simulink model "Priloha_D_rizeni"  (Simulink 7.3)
settings: Solver=ode45  StartTime=0.0  StopTime=0.7  FixedStep=0.6e-3  MaxStep=0.08e-3  RelTol=0.8e-3
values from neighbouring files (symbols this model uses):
  ILi = [0 Imax]    [Priloha_B_motor1_parametry.m]    (also in Priloha_C_motor2_parametry.m)
  Im = Psim / Ldi(1)    [Priloha_B_motor1_parametry.m]    (also in Priloha_C_motor2_parametry.m)
  Imax = 8    [Priloha_B_motor1_parametry.m]    (also in Priloha_C_motor2_parametry.m)
  J = 7e-3    (= 0.007)    [Priloha_B_motor1_parametry.m]    (also in Priloha_C_motor2_parametry.m)
  Kiid = 1 / (KM * 2 * tausigmaid / Rs)    (= 1975)    [Priloha_B_motor1_parametry.m]    (also in Priloha_C_motor2_parametry.m)
  Kiiq = 1 / (KM * 2 * tausigmaiq / Rs)    (= 1975)    [Priloha_B_motor1_parametry.m]    (also in Priloha_C_motor2_parametry.m)
  Kiwq = 1 / (Psim * p * 8 * (2 * tausigmaiq)^2 / J)    (= 306.115309264)    [Priloha_B_motor1_parametry.m]    (also in Priloha_C_motor2_parametry.m = 402.854511971)
  KM = 1    [Priloha_B_motor1_parametry.m]    (also in Priloha_C_motor2_parametry.m)
  Kpid = Ldi(1) / (KM * 2 * tausigmaid)    [Priloha_B_motor1_parametry.m]    (also in Priloha_C_motor2_parametry.m)
  Kpiq = Lqi(1) / (KM * 2 * tausigmaiq)    [Priloha_B_motor1_parametry.m]    (also in Priloha_C_motor2_parametry.m)
  Kpwq = 4 / (Psim * p * 8 * (2 * tausigmaiq) / J)    (= 2.44892247411)    [Priloha_B_motor1_parametry.m]    (also in Priloha_C_motor2_parametry.m = 3.22283609576)
  Ld = 22.5e-3    (= 0.0225)    [Priloha_B_motor1_parametry.m]    (also in Priloha_C_motor2_parametry.m)
  Ldi = [Ldi Ldi]    [Priloha_B_motor1_parametry.m]    (also in Priloha_C_motor2_parametry.m)
  Lq = 54e-3    (= 0.054)    [Priloha_B_motor1_parametry.m]    (also in Priloha_C_motor2_parametry.m)
  Lqi = [Lqi Lqi]    [Priloha_B_motor1_parametry.m]    (also in Priloha_C_motor2_parametry.m)
  p = 3    [Priloha_B_motor1_parametry.m]    (also in Priloha_C_motor2_parametry.m)
  Psim = 238.2e-3    (= 0.2382)    [Priloha_B_motor1_parametry.m]    (also in Priloha_C_motor2_parametry.m = 0.181)
  Rs = 3.95    [Priloha_B_motor1_parametry.m]    (also in Priloha_C_motor2_parametry.m)
  tausigmaid = 1 / fM    (= 0.001)    [Priloha_B_motor1_parametry.m]    (also in Priloha_C_motor2_parametry.m)
  tausigmaiq = 1 / fM    (= 0.001)    [Priloha_B_motor1_parametry.m]    (also in Priloha_C_motor2_parametry.m)
  Umax = 115    [Priloha_B_motor1_parametry.m]    (also in Priloha_C_motor2_parametry.m)
undefined symbols (not defined in the file or in its folder): Floor, magnitude
libraries: simulink x21
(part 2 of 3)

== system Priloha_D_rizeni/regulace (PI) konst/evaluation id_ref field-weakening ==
  note: PI-regulator napeti
  us : Inport
  id_mtpa : Inport  Port=2
  Add : Sum  OutDataType=fixdt(1, 16)  OutScaling=2^-10
  Add3 : Sum  Inputs=+-  OutDataType=fixdt(1, 16)  OutScaling=2^-10
  Compare To Constant : simulink/Logic and Bit Operations/Compare To Constant  SystemSampleTime=-1  relop=<  const=Umax * 0.98  LogicOutDataTypeMode=boolean
  I : Gain  Gain=10  ParameterDataType=fixdt(1, 16)  ParameterScaling=2^0  OutDataType=fixdt(1, 16)  OutScaling=2^0
  Integrator1 : Integrator  ExternalReset=level  InitialConditionSource=external  LimitOutput=on  UpperSaturationLimit=Imax  LowerSaturationLimit=-Imax
  P2 : Gain  Gain=0.08  ParameterDataType=fixdt(1, 16)  ParameterScaling=2^0  OutDataType=fixdt(1, 16)  OutScaling=2^0
  Saturation Dynamic : Subsystem  AncestorBlock=simulink/Discontinuities/Saturation Dynamic  mask(Saturation Dynamic){OutMin=[], OutMax=[], OutDataTypeStr=Inherit: Same as second input, OutputDataTypeScalingMode=Same as second input, OutDataType=fixdt(1, 16), OutScaling=2^-10, LockScale=off, RndMeth=Floor, DoSatur=off}
      mask prompts: OutMin "Output minimum:"; OutMax "Output maximum:"; OutDataTypeStr "Output data type:"; OutputDataTypeScalingMode "Output data type mode:"; OutDataType "Output data type (e.g. fixdt(1, 16), fixdt('single')):"; OutScaling "Output scaling (Slope, e.g. 2^-9 or [Slope Bias], e.g. [1.25 3]):"; LockScale "Lock output scaling against changes by the autoscaling tool"; RndMeth "Integer rounding mode:"; DoSatur "Saturate on integer overflow"
      mask help: Bound the range of the second input by using the first input (upper limit) and the third input (lower limit).
      mask init:
      | blkH = gcbh;
      | blkName = getfullname(blkH);
      | 
      | switch_blks = {'Switch','Switch2'}; 
      | for i = 1:length(switch_blks)
      |   set_param([blkName,'/',switch_blks{i}], ...
      |       'RndMeth', RndMeth, ...
      | 	  'DoSatur', DoSatur);
      | end
      | 
      | propBlk = [blkName, '/Data Type Propagation'];
      | 
      | if strcmp(OutputDataTypeScalingMode, 'Same as second input')
      |     set_param(propBlk, 'PropDataTypeMode', 'Inherit via propagation rule', ...
      |                        'PropScalingMode',  'Inherit via propagation rule');
      | else
      |     scaling = OutScaling;
      |     switch OutputDataTypeScalingMode
      |       case 'double'
      |         dataType = 'fixdt(''double'')';
      |       case 'single'
      |         dataType = 'fixdt(''single'')';
      |       case 'int8'
      |         dataType = 'fixdt(1,8,0)';
      |       case 'uint8'
      |         dataType = 'fixdt(0,8,0)';
      |       case 'int16'
      |         dataType = 'fixdt(1,16,0)';
      |       case 'uint16'
      |         dataType = 'fixdt(0,16,0)';
      |       case 'int32'
      |         dataType = 'fixdt(1,32,0)';
      |       case 'uint32'
      |         dataType = 'fixdt(0,32,0)';
      |       case 'Specify via dialog'
      |         dataType = OutDataType;
      |     end
      |     
      |     set_param(propBlk, 'PropDataTypeMode', 'Specify via dialog', ...
      |                        'PropScalingMode',  'Specify via dialog', ...
      |                        'PropDataType',     dataType, ...
      |                        'PropScaling',      scaling);
      | end
  id_ref1 : Constant  Value=100  OutDataType=fixdt(1, 16)  OutScaling=2^0
  id_ref2 : Constant  Value=0  OutDataType=fixdt(1, 16)  OutScaling=2^0
  id_ref4 : Constant  Value=-Imax  OutDataType=fixdt(1, 16)  OutScaling=2^0
  id_ref : Outport
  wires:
  id_ref1/1 -> Add3/1
  us/1 -> Add3/2, Compare To Constant/1
  Add/1 -> Saturation Dynamic/2(u)
  Add3/1 -> P2/1, I/1
  id_ref2/1 -> Saturation Dynamic/1(up)
  id_ref4/1 -> Saturation Dynamic/3(lo)
  Compare To Constant/1 -> Integrator1/2
  Saturation Dynamic/1(y1) -> id_ref/1
  I/1 -> Integrator1/1
  P2/1 -> Add/1
  Integrator1/1 -> Add/2
  id_mtpa/1 -> Integrator1/3

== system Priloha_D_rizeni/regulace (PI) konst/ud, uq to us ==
  ud2 : Inport
  uq2 : Inport  Port=2
  Add3 : Sum  OutDataType=fixdt(1, 16)  OutScaling=2^-10
  Math Function : Math  Operator=magnitude^2  OutputSignalType=real  OutDataType=fixdt(1, 16)  OutScaling=2^0
  Math Function1 : Math  Operator=magnitude^2  OutputSignalType=real  OutDataType=fixdt(1, 16)  OutScaling=2^0
  Math Funtion2 : Math  Operator=sqrt  OutputSignalType=real  OutDataType=fixdt(1, 16)  OutScaling=2^0
  us : Outport
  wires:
  Math Function/1 -> Add3/1
  Math Function1/1 -> Add3/2
  Add3/1 -> Math Funtion2/1
  ud2/1 -> Math Function/1
  Math Funtion2/1 -> us/1
  uq2/1 -> Math Function1/1

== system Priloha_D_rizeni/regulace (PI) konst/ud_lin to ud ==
  ud1 : Inport
  wm : Inport  Port=2
  iq : Inport  Port=3
  Add6 : Sum  Inputs=+-  OutDataType=fixdt(1, 16)  OutScaling=2^-10
  Gain1 : Gain  Gain=p  ParameterDataType=fixdt(1, 16)  ParameterScaling=2^0  OutDataType=fixdt(1, 16)  OutScaling=2^0
  Gain2 : Gain  Gain=Lq  ParameterDataType=fixdt(1, 16)  ParameterScaling=2^0  OutDataType=fixdt(1, 16)  OutScaling=2^0
  Product6 : Product  OutDataType=fixdt(1, 16)  OutScaling=2^0
  ud2 : Outport
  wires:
  Gain1/1 -> Product6/1
  Product6/1 -> Add6/2
  Add6/1 -> ud2/1
  wm/1 -> Gain1/1
  ud1/1 -> Add6/1
  Gain2/1 -> Product6/2
  iq/1 -> Gain2/1

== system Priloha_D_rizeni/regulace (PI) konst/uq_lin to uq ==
  uq1 : Inport
  wm : Inport  Port=2
  id : Inport  Port=3
  Add1 : Sum  OutDataType=fixdt(1, 16)  OutScaling=2^-10
  Add2 : Sum  OutDataType=fixdt(1, 16)  OutScaling=2^-10
  Gain1 : Gain  Gain=Ld  ParameterDataType=fixdt(1, 16)  ParameterScaling=2^0  OutDataType=fixdt(1, 16)  OutScaling=2^0
  Gain2 : Gain  Gain=p  ParameterDataType=fixdt(1, 16)  ParameterScaling=2^0  OutDataType=fixdt(1, 16)  OutScaling=2^0
  Product1 : Product  OutDataType=fixdt(1, 16)  OutScaling=2^0
  id_ref1 : Constant  Value=Ld * Im  OutDataType=fixdt(1, 16)  OutScaling=2^0
  uq2 : Outport
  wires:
  Product1/1 -> Add1/2
  Gain2/1 -> Product1/1
  Add1/1 -> uq2/1
  wm/1 -> Gain2/1
  uq1/1 -> Add1/1
  Add2/1 -> Product1/2
  id/1 -> Gain1/1
  Gain1/1 -> Add2/1
  id_ref1/1 -> Add2/2

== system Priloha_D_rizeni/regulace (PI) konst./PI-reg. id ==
  note: PI-regulator proudu id
  id_ref : Inport
  id : Inport  Port=2
  Add : Sum  OutDataType=fixdt(1, 16)  OutScaling=2^-10
  Add1 : Sum  Inputs=+-  OutDataType=fixdt(1, 16)  OutScaling=2^-10
  I : Gain  Gain=Kiid  ParameterDataType=fixdt(1, 16)  ParameterScaling=2^0  OutDataType=fixdt(1, 16)  OutScaling=2^0
  Integrator1 : Integrator  LimitOutput=on  UpperSaturationLimit=Umax  LowerSaturationLimit=-Umax
  P2 : Gain  Gain=Kpid  ParameterDataType=fixdt(1, 16)  ParameterScaling=2^0  OutDataType=fixdt(1, 16)  OutScaling=2^0
  ud1 : Outport
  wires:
  P2/1 -> Add/1
  Integrator1/1 -> Add/2
  id_ref/1 -> Add1/1
  id/1 -> Add1/2
  I/1 -> Integrator1/1
  Add1/1 -> I/1, P2/1
  Add/1 -> ud1/1

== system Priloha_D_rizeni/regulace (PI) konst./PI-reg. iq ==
  note: PI-regulator proudu iq
  iq_ref : Inport
  iq : Inport  Port=2
  Add : Sum  OutDataType=fixdt(1, 16)  OutScaling=2^-10
  Add1 : Sum  Inputs=+-  OutDataType=fixdt(1, 16)  OutScaling=2^-10
  I : Gain  Gain=Kiiq  ParameterDataType=fixdt(1, 16)  ParameterScaling=2^0  OutDataType=fixdt(1, 16)  OutScaling=2^0
  Integrator1 : Integrator  LimitOutput=on  UpperSaturationLimit=Umax  LowerSaturationLimit=-Umax
  P : Gain  Gain=Kpiq  ParameterDataType=fixdt(1, 16)  ParameterScaling=2^0  OutDataType=fixdt(1, 16)  OutScaling=2^0
  uq1 : Outport
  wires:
  Integrator1/1 -> Add/2
  P/1 -> Add/1
  iq_ref/1 -> Add1/1
  iq/1 -> Add1/2
  Add/1 -> uq1/1
  I/1 -> Integrator1/1
  Add1/1 -> P/1, I/1

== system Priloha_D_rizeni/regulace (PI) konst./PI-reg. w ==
  note: PI-regulator otacek
  w_ref : Inport
  wm : Inport  Port=2
  id_ref : Inport  Port=3
  Add : Sum  OutDataType=fixdt(1, 16)  OutScaling=2^-10
  Add2 : Sum  Inputs=+-  OutDataType=fixdt(1, 16)  OutScaling=2^-10
  Add3 : Sum  Inputs=+-  OutDataType=fixdt(1, 16)  OutScaling=2^-10
  I : Gain  Gain=Kiwq  ParameterDataType=fixdt(1, 16)  ParameterScaling=2^0  OutDataType=fixdt(1, 16)  OutScaling=2^0
  I1 : Gain  Gain=-1  ParameterDataType=fixdt(1, 16)  ParameterScaling=2^0  OutDataType=fixdt(1, 16)  OutScaling=2^0
  Integrator1 : Integrator  LimitOutput=on  UpperSaturationLimit=Imax  LowerSaturationLimit=-Imax
  Math Function : Math  Operator=magnitude^2  OutputSignalType=real  OutDataType=fixdt(1, 16)  OutScaling=2^0
  Math Funtion2 : Math  Operator=sqrt  OutputSignalType=real  OutDataType=fixdt(1, 16)  OutScaling=2^0
  P : Gain  Gain=Kpwq  ParameterDataType=fixdt(1, 16)  ParameterScaling=2^0  OutDataType=fixdt(1, 16)  OutScaling=2^0
  Saturation Dynamic : Subsystem  AncestorBlock=simulink/Discontinuities/Saturation Dynamic  mask(Saturation Dynamic){OutMin=[], OutMax=[], OutDataTypeStr=Inherit: Same as second input, OutputDataTypeScalingMode=Same as second input, OutDataType=fixdt(1, 16), OutScaling=2^-10, LockScale=off, RndMeth=Floor, DoSatur=off}
      mask prompts: OutMin "Output minimum:"; OutMax "Output maximum:"; OutDataTypeStr "Output data type:"; OutputDataTypeScalingMode "Output data type mode:"; OutDataType "Output data type (e.g. fixdt(1, 16), fixdt('single')):"; OutScaling "Output scaling (Slope, e.g. 2^-9 or [Slope Bias], e.g. [1.25 3]):"; LockScale "Lock output scaling against changes by the autoscaling tool"; RndMeth "Integer rounding mode:"; DoSatur "Saturate on integer overflow"
      mask help: Bound the range of the second input by using the first input (upper limit) and the third input (lower limit).
      mask init:
      | blkH = gcbh;
      | blkName = getfullname(blkH);
      | 
      | switch_blks = {'Switch','Switch2'}; 
      | for i = 1:length(switch_blks)
      |   set_param([blkName,'/',switch_blks{i}], ...
      |       'RndMeth', RndMeth, ...
      | 	  'DoSatur', DoSatur);
      | end
      | 
      | propBlk = [blkName, '/Data Type Propagation'];
      | 
      | if strcmp(OutputDataTypeScalingMode, 'Same as second input')
      |     set_param(propBlk, 'PropDataTypeMode', 'Inherit via propagation rule', ...
      |                        'PropScalingMode',  'Inherit via propagation rule');
      | else
      |     scaling = OutScaling;
      |     switch OutputDataTypeScalingMode
      |       case 'double'
      |         dataType = 'fixdt(''double'')';
      |       case 'single'
      |         dataType = 'fixdt(''single'')';
      |       case 'int8'
      |         dataType = 'fixdt(1,8,0)';
      |       case 'uint8'
      |         dataType = 'fixdt(0,8,0)';
      |       case 'int16'
      |         dataType = 'fixdt(1,16,0)';
      |       case 'uint16'
      |         dataType = 'fixdt(0,16,0)';
      |       case 'int32'
      |         dataType = 'fixdt(1,32,0)';
      |       case 'uint32'
      |         dataType = 'fixdt(0,32,0)';
      |       case 'Specify via dialog'
      |         dataType = OutDataType;
      |     end
      |     
      |     set_param(propBlk, 'PropDataTypeMode', 'Specify via dialog', ...
      |                        'PropScalingMode',  'Specify via dialog', ...
      |                        'PropDataType',     dataType, ...
      |                        'PropScaling',      scaling);
      | end
  id_ref4 : Constant  Value=Imax^2  OutDataType=fixdt(1, 16)  OutScaling=2^0
  iq_ref : Outport
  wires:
  P/1 -> Add/1
  Integrator1/1 -> Add/2
  Add/1 -> Saturation Dynamic/2(u)
  w_ref/1 -> Add2/1
  wm/1 -> Add2/2
  Add2/1 -> P/1, I/1
  Saturation Dynamic/1(y1) -> iq_ref/1
  I/1 -> Integrator1/1
  id_ref/1 -> Math Function/1
  Add3/1 -> Math Funtion2/1
  Math Funtion2/1 -> Saturation Dynamic/1(up), I1/1
  Math Function/1 -> Add3/2
  id_ref4/1 -> Add3/1
  I1/1 -> Saturation Dynamic/3(lo)

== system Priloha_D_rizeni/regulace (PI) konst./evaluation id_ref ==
  iq_ref : Inport
  Add3 : Sum  OutDataType=fixdt(1, 16)  OutScaling=2^-10
  Add4 : Sum  Inputs=+-  OutDataType=fixdt(1, 16)  OutScaling=2^-10
  Divide : Product  Inputs=*/  OutDataType=fixdt(1, 16)  OutScaling=2^-10
  Divide1 : Product  Inputs=*/  OutDataType=fixdt(1, 16)  OutScaling=2^-10
  Gain : Gain  Gain=4  ParameterDataType=fixdt(1, 16)  ParameterScaling=2^0  OutDataType=fixdt(1, 16)  OutScaling=2^0
  Gain1 : Gain  Gain=2  ParameterDataType=fixdt(1, 16)  ParameterScaling=2^0  OutDataType=fixdt(1, 16)  OutScaling=2^0
  Math Function : Math  Operator=magnitude^2  OutputSignalType=real  OutDataType=fixdt(1, 16)  OutScaling=2^0
  Math Function1 : Math  Operator=magnitude^2  OutputSignalType=real  OutDataType=fixdt(1, 16)  OutScaling=2^0
  Math Function2 : Math  Operator=magnitude^2  OutputSignalType=real  OutDataType=fixdt(1, 16)  OutScaling=2^0
  Math Function3 : Math  Operator=sqrt  OutputSignalType=real  OutDataType=fixdt(1, 16)  OutScaling=2^0
  w_ref1 : Constant  Value=Lq - Ld  OutDataType=fixdt(1, 16)  OutScaling=2^0
  w_ref2 : Constant  Value=Psim  OutDataType=fixdt(1, 16)  OutScaling=2^0
  id_ref : Outport
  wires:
  Math Function/1 -> Add3/2
  w_ref2/1 -> Math Function1/1, Divide1/1
  Math Function1/1 -> Divide/1
  Math Function2/1 -> Gain/1
  Divide/1 -> Add3/1
  Add3/1 -> Math Function3/1
  Divide1/1 -> Add4/1
  w_ref1/1 -> Math Function2/1, Gain1/1
  Math Function3/1 -> Add4/2
  Gain/1 -> Divide/2
  Gain1/1 -> Divide1/2
  iq_ref/1 -> Math Function/1
  Add4/1 -> id_ref/1

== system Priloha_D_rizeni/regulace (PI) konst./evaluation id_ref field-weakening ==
  note: PI-regulator napeti
  us : Inport
  id_mtpa : Inport  Port=2
  Add : Sum  OutDataType=fixdt(1, 16)  OutScaling=2^-10
  Add3 : Sum  Inputs=+-  OutDataType=fixdt(1, 16)  OutScaling=2^-10
  Compare To Constant : simulink/Logic and Bit Operations/Compare To Constant  SystemSampleTime=-1  relop=<  const=Umax * 0.98  LogicOutDataTypeMode=boolean
  I : Gain  Gain=10  ParameterDataType=fixdt(1, 16)  ParameterScaling=2^0  OutDataType=fixdt(1, 16)  OutScaling=2^0
  Integrator1 : Integrator  ExternalReset=level  InitialConditionSource=external  LimitOutput=on  UpperSaturationLimit=Imax  LowerSaturationLimit=-Imax
  P2 : Gain  Gain=0.08  ParameterDataType=fixdt(1, 16)  ParameterScaling=2^0  OutDataType=fixdt(1, 16)  OutScaling=2^0
  Saturation Dynamic : Subsystem  AncestorBlock=simulink/Discontinuities/Saturation Dynamic  mask(Saturation Dynamic){OutMin=[], OutMax=[], OutDataTypeStr=Inherit: Same as second input, OutputDataTypeScalingMode=Same as second input, OutDataType=fixdt(1, 16), OutScaling=2^-10, LockScale=off, RndMeth=Floor, DoSatur=off}
      mask prompts: OutMin "Output minimum:"; OutMax "Output maximum:"; OutDataTypeStr "Output data type:"; OutputDataTypeScalingMode "Output data type mode:"; OutDataType "Output data type (e.g. fixdt(1, 16), fixdt('single')):"; OutScaling "Output scaling (Slope, e.g. 2^-9 or [Slope Bias], e.g. [1.25 3]):"; LockScale "Lock output scaling against changes by the autoscaling tool"; RndMeth "Integer rounding mode:"; DoSatur "Saturate on integer overflow"
      mask help: Bound the range of the second input by using the first input (upper limit) and the third input (lower limit).
      mask init:
      | blkH = gcbh;
      | blkName = getfullname(blkH);
      | 
      | switch_blks = {'Switch','Switch2'}; 
      | for i = 1:length(switch_blks)
      |   set_param([blkName,'/',switch_blks{i}], ...
      |       'RndMeth', RndMeth, ...
      | 	  'DoSatur', DoSatur);
      | end
      | 
      | propBlk = [blkName, '/Data Type Propagation'];
      | 
      | if strcmp(OutputDataTypeScalingMode, 'Same as second input')
      |     set_param(propBlk, 'PropDataTypeMode', 'Inherit via propagation rule', ...
      |                        'PropScalingMode',  'Inherit via propagation rule');
      | else
      |     scaling = OutScaling;
      |     switch OutputDataTypeScalingMode
      |       case 'double'
      |         dataType = 'fixdt(''double'')';
      |       case 'single'
      |         dataType = 'fixdt(''single'')';
      |       case 'int8'
      |         dataType = 'fixdt(1,8,0)';
      |       case 'uint8'
      |         dataType = 'fixdt(0,8,0)';
      |       case 'int16'
      |         dataType = 'fixdt(1,16,0)';
      |       case 'uint16'
      |         dataType = 'fixdt(0,16,0)';
      |       case 'int32'
      |         dataType = 'fixdt(1,32,0)';
      |       case 'uint32'
      |         dataType = 'fixdt(0,32,0)';
      |       case 'Specify via dialog'
      |         dataType = OutDataType;
      |     end
      |     
      |     set_param(propBlk, 'PropDataTypeMode', 'Specify via dialog', ...
      |                        'PropScalingMode',  'Specify via dialog', ...
      |                        'PropDataType',     dataType, ...
      |                        'PropScaling',      scaling);
      | end
  id_ref1 : Constant  Value=100  OutDataType=fixdt(1, 16)  OutScaling=2^0
  id_ref2 : Constant  Value=0  OutDataType=fixdt(1, 16)  OutScaling=2^0
  id_ref4 : Constant  Value=-Imax  OutDataType=fixdt(1, 16)  OutScaling=2^0
  id_ref : Outport
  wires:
  id_ref1/1 -> Add3/1
  us/1 -> Add3/2, Compare To Constant/1
  Add/1 -> Saturation Dynamic/2(u)
  Add3/1 -> P2/1, I/1
  id_ref2/1 -> Saturation Dynamic/1(up)
  id_ref4/1 -> Saturation Dynamic/3(lo)
  Compare To Constant/1 -> Integrator1/2
  Saturation Dynamic/1(y1) -> id_ref/1
  I/1 -> Integrator1/1
  P2/1 -> Add/1
  Integrator1/1 -> Add/2
  id_mtpa/1 -> Integrator1/3

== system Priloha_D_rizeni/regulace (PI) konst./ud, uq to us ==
  ud1 : Inport
  uq1 : Inport  Port=2
  Add3 : Sum  OutDataType=fixdt(1, 16)  OutScaling=2^-10
  Math Function : Math  Operator=magnitude^2  OutputSignalType=real  OutDataType=fixdt(1, 16)  OutScaling=2^0
  Math Function1 : Math  Operator=magnitude^2  OutputSignalType=real  OutDataType=fixdt(1, 16)  OutScaling=2^0
  Math Funtion2 : Math  Operator=sqrt  OutputSignalType=real  OutDataType=fixdt(1, 16)  OutScaling=2^0
  us : Outport
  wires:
  Math Function/1 -> Add3/1
  Math Function1/1 -> Add3/2
  Add3/1 -> Math Funtion2/1
  ud1/1 -> Math Function/1
  Math Funtion2/1 -> us/1
  uq1/1 -> Math Function1/1

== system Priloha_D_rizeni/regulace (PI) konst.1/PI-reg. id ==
  note: PI-regulator proudu id
  id_ref : Inport
  id : Inport  Port=2
  Add : Sum  OutDataType=fixdt(1, 16)  OutScaling=2^-10
  Add1 : Sum  Inputs=+-  OutDataType=fixdt(1, 16)  OutScaling=2^-10
  I : Gain  Gain=Kiid  ParameterDataType=fixdt(1, 16)  ParameterScaling=2^0  OutDataType=fixdt(1, 16)  OutScaling=2^0
  Integrator1 : Integrator  LimitOutput=on  UpperSaturationLimit=Umax  LowerSaturationLimit=-Umax
  P2 : Gain  Gain=Kpid  ParameterDataType=fixdt(1, 16)  ParameterScaling=2^0  OutDataType=fixdt(1, 16)  OutScaling=2^0
  Saturation3 : Saturate  UpperLimit=Umax  LowerLimit=-Umax  OutDataType=fixdt(1, 16)  OutScaling=2^0
  Saturation5 : Saturate  UpperLimit=Umax  LowerLimit=-Umax  OutDataType=fixdt(1, 16)  OutScaling=2^0
  ud1 : Outport
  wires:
  P2/1 -> Saturation3/1
  Integrator1/1 -> Add/2
  Add/1 -> Saturation5/1
  id_ref/1 -> Add1/1
  id/1 -> Add1/2
  I/1 -> Integrator1/1
  Add1/1 -> I/1, P2/1
  Saturation3/1 -> Add/1
  Saturation5/1 -> ud1/1

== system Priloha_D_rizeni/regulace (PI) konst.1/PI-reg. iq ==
  note: PI-regulator proudu iq
  iq_ref : Inport
  iq : Inport  Port=2
  Add : Sum  OutDataType=fixdt(1, 16)  OutScaling=2^-10
  Add1 : Sum  Inputs=+-  OutDataType=fixdt(1, 16)  OutScaling=2^-10
  I : Gain  Gain=Kiiq  ParameterDataType=fixdt(1, 16)  ParameterScaling=2^0  OutDataType=fixdt(1, 16)  OutScaling=2^0
  Integrator1 : Integrator  LimitOutput=on  UpperSaturationLimit=Umax  LowerSaturationLimit=-Umax
  P : Gain  Gain=Kpiq  ParameterDataType=fixdt(1, 16)  ParameterScaling=2^0  OutDataType=fixdt(1, 16)  OutScaling=2^0
  Saturation2 : Saturate  UpperLimit=Umax  LowerLimit=-Umax  OutDataType=fixdt(1, 16)  OutScaling=2^0
  Saturation3 : Saturate  UpperLimit=Umax  LowerLimit=-Umax  OutDataType=fixdt(1, 16)  OutScaling=2^0
  uq1 : Outport
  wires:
  Integrator1/1 -> Add/2
  P/1 -> Saturation2/1
  iq_ref/1 -> Add1/1
  iq/1 -> Add1/2
  Add/1 -> Saturation3/1
  I/1 -> Integrator1/1
  Add1/1 -> P/1, I/1
  Saturation2/1 -> Add/1
  Saturation3/1 -> uq1/1

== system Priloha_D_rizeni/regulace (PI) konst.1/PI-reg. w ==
  note: PI-regulator otacek
  w_ref : Inport
  wm : Inport  Port=2
  id_ref : Inport  Port=3
  Add : Sum  OutDataType=fixdt(1, 16)  OutScaling=2^-10
  Add2 : Sum  Inputs=+-  OutDataType=fixdt(1, 16)  OutScaling=2^-10
  Add3 : Sum  Inputs=+-  OutDataType=fixdt(1, 16)  OutScaling=2^-10
  I : Gain  Gain=Kiwq  ParameterDataType=fixdt(1, 16)  ParameterScaling=2^0  OutDataType=fixdt(1, 16)  OutScaling=2^0
  I1 : Gain  Gain=-1  ParameterDataType=fixdt(1, 16)  ParameterScaling=2^0  OutDataType=fixdt(1, 16)  OutScaling=2^0
  Integrator1 : Integrator  LimitOutput=on  UpperSaturationLimit=Imax  LowerSaturationLimit=-Imax
  Math Function : Math  Operator=magnitude^2  OutputSignalType=real  OutDataType=fixdt(1, 16)  OutScaling=2^0
  Math Funtion2 : Math  Operator=sqrt  OutputSignalType=real  OutDataType=fixdt(1, 16)  OutScaling=2^0
  P : Gain  Gain=Kpwq  ParameterDataType=fixdt(1, 16)  ParameterScaling=2^0  OutDataType=fixdt(1, 16)  OutScaling=2^0
  Saturation Dynamic : Subsystem  AncestorBlock=simulink/Discontinuities/Saturation Dynamic  mask(Saturation Dynamic){OutMin=[], OutMax=[], OutDataTypeStr=Inherit: Same as second input, OutputDataTypeScalingMode=Same as second input, OutDataType=fixdt(1, 16), OutScaling=2^-10, LockScale=off, RndMeth=Floor, DoSatur=off}
      mask prompts: OutMin "Output minimum:"; OutMax "Output maximum:"; OutDataTypeStr "Output data type:"; OutputDataTypeScalingMode "Output data type mode:"; OutDataType "Output data type (e.g. fixdt(1, 16), fixdt('single')):"; OutScaling "Output scaling (Slope, e.g. 2^-9 or [Slope Bias], e.g. [1.25 3]):"; LockScale "Lock output scaling against changes by the autoscaling tool"; RndMeth "Integer rounding mode:"; DoSatur "Saturate on integer overflow"
      mask help: Bound the range of the second input by using the first input (upper limit) and the third input (lower limit).
      mask init:
      | blkH = gcbh;
      | blkName = getfullname(blkH);
      | 
      | switch_blks = {'Switch','Switch2'}; 
      | for i = 1:length(switch_blks)
      |   set_param([blkName,'/',switch_blks{i}], ...
      |       'RndMeth', RndMeth, ...
      | 	  'DoSatur', DoSatur);
      | end
      | 
      | propBlk = [blkName, '/Data Type Propagation'];
      | 
      | if strcmp(OutputDataTypeScalingMode, 'Same as second input')
      |     set_param(propBlk, 'PropDataTypeMode', 'Inherit via propagation rule', ...
      |                        'PropScalingMode',  'Inherit via propagation rule');
      | else
      |     scaling = OutScaling;
      |     switch OutputDataTypeScalingMode
      |       case 'double'
      |         dataType = 'fixdt(''double'')';
      |       case 'single'
      |         dataType = 'fixdt(''single'')';
      |       case 'int8'
      |         dataType = 'fixdt(1,8,0)';
      |       case 'uint8'
      |         dataType = 'fixdt(0,8,0)';
      |       case 'int16'
      |         dataType = 'fixdt(1,16,0)';
      |       case 'uint16'
      |         dataType = 'fixdt(0,16,0)';
      |       case 'int32'
      |         dataType = 'fixdt(1,32,0)';
      |       case 'uint32'
      |         dataType = 'fixdt(0,32,0)';
      |       case 'Specify via dialog'
      |         dataType = OutDataType;
      |     end
      |     
      |     set_param(propBlk, 'PropDataTypeMode', 'Specify via dialog', ...
      |                        'PropScalingMode',  'Specify via dialog', ...
      |                        'PropDataType',     dataType, ...
      |                        'PropScaling',      scaling);
      | end
  id_ref4 : Constant  Value=Imax^2  OutDataType=fixdt(1, 16)  OutScaling=2^0
  iq_ref : Outport
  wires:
  P/1 -> Add/1
  Integrator1/1 -> Add/2
  Add/1 -> Saturation Dynamic/2(u)
  w_ref/1 -> Add2/1
  wm/1 -> Add2/2
  Add2/1 -> P/1, I/1
  Saturation Dynamic/1(y1) -> iq_ref/1
  I/1 -> Integrator1/1
  id_ref/1 -> Math Function/1
  Add3/1 -> Math Funtion2/1
  Math Funtion2/1 -> Saturation Dynamic/1(up), I1/1
  Math Function/1 -> Add3/2
  id_ref4/1 -> Add3/1
  I1/1 -> Saturation Dynamic/3(lo)

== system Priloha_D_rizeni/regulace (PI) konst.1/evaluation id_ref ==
  iq_ref : Inport
  Add3 : Sum  OutDataType=fixdt(1, 16)  OutScaling=2^-10
  Add4 : Sum  Inputs=+-  OutDataType=fixdt(1, 16)  OutScaling=2^-10
  Divide : Product  Inputs=*/  OutDataType=fixdt(1, 16)  OutScaling=2^-10
  Divide1 : Product  Inputs=*/  OutDataType=fixdt(1, 16)  OutScaling=2^-10
  Gain : Gain  Gain=4  ParameterDataType=fixdt(1, 16)  ParameterScaling=2^0  OutDataType=fixdt(1, 16)  OutScaling=2^0
  Gain1 : Gain  Gain=2  ParameterDataType=fixdt(1, 16)  ParameterScaling=2^0  OutDataType=fixdt(1, 16)  OutScaling=2^0
  Math Function : Math  Operator=magnitude^2  OutputSignalType=real  OutDataType=fixdt(1, 16)  OutScaling=2^0
  Math Function1 : Math  Operator=magnitude^2  OutputSignalType=real  OutDataType=fixdt(1, 16)  OutScaling=2^0
  Math Function2 : Math  Operator=magnitude^2  OutputSignalType=real  OutDataType=fixdt(1, 16)  OutScaling=2^0
  Math Function3 : Math  Operator=sqrt  OutputSignalType=real  OutDataType=fixdt(1, 16)  OutScaling=2^0
  w_ref1 : Constant  Value=Lq - Ld  OutDataType=fixdt(1, 16)  OutScaling=2^0
  w_ref2 : Constant  Value=Psim  OutDataType=fixdt(1, 16)  OutScaling=2^0
  id_ref : Outport
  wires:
  Math Function/1 -> Add3/2
  w_ref2/1 -> Math Function1/1, Divide1/1
  Math Function1/1 -> Divide/1
  Math Function2/1 -> Gain/1
  Divide/1 -> Add3/1
  Add3/1 -> Math Function3/1
  Divide1/1 -> Add4/1
  w_ref1/1 -> Math Function2/1, Gain1/1
  Math Function3/1 -> Add4/2
  Gain/1 -> Divide/2
  Gain1/1 -> Divide1/2
  iq_ref/1 -> Math Function/1
  Add4/1 -> id_ref/1

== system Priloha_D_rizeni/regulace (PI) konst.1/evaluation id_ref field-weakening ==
  note: PI-regulator napeti
  us : Inport
  id_mtpa : Inport  Port=2
  Add : Sum  OutDataType=fixdt(1, 16)  OutScaling=2^-10
  Add3 : Sum  Inputs=+-  OutDataType=fixdt(1, 16)  OutScaling=2^-10
  Compare To Constant : simulink/Logic and Bit Operations/Compare To Constant  SystemSampleTime=-1  relop=<  const=Umax * 0.92  LogicOutDataTypeMode=boolean
  I : Gain  Gain=10  ParameterDataType=fixdt(1, 16)  ParameterScaling=2^0  OutDataType=fixdt(1, 16)  OutScaling=2^0
  Integrator1 : Integrator  ExternalReset=level  InitialConditionSource=external  LimitOutput=on  UpperSaturationLimit=Imax  LowerSaturationLimit=-Imax
  P2 : Gain  Gain=0.08  ParameterDataType=fixdt(1, 16)  ParameterScaling=2^0  OutDataType=fixdt(1, 16)  OutScaling=2^0
  Saturation Dynamic : Subsystem  AncestorBlock=simulink/Discontinuities/Saturation Dynamic  mask(Saturation Dynamic){OutMin=[], OutMax=[], OutDataTypeStr=Inherit: Same as second input, OutputDataTypeScalingMode=Same as second input, OutDataType=fixdt(1, 16), OutScaling=2^-10, LockScale=off, RndMeth=Floor, DoSatur=off}
      mask prompts: OutMin "Output minimum:"; OutMax "Output maximum:"; OutDataTypeStr "Output data type:"; OutputDataTypeScalingMode "Output data type mode:"; OutDataType "Output data type (e.g. fixdt(1, 16), fixdt('single')):"; OutScaling "Output scaling (Slope, e.g. 2^-9 or [Slope Bias], e.g. [1.25 3]):"; LockScale "Lock output scaling against changes by the autoscaling tool"; RndMeth "Integer rounding mode:"; DoSatur "Saturate on integer overflow"
      mask help: Bound the range of the second input by using the first input (upper limit) and the third input (lower limit).
      mask init:
      | blkH = gcbh;
      | blkName = getfullname(blkH);
      | 
      | switch_blks = {'Switch','Switch2'}; 
      | for i = 1:length(switch_blks)
      |   set_param([blkName,'/',switch_blks{i}], ...
      |       'RndMeth', RndMeth, ...
      | 	  'DoSatur', DoSatur);
      | end
      | 
      | propBlk = [blkName, '/Data Type Propagation'];
      | 
      | if strcmp(OutputDataTypeScalingMode, 'Same as second input')
      |     set_param(propBlk, 'PropDataTypeMode', 'Inherit via propagation rule', ...
      |                        'PropScalingMode',  'Inherit via propagation rule');
      | else
      |     scaling = OutScaling;
      |     switch OutputDataTypeScalingMode
      |       case 'double'
      |         dataType = 'fixdt(''double'')';
      |       case 'single'
      |         dataType = 'fixdt(''single'')';
      |       case 'int8'
      |         dataType = 'fixdt(1,8,0)';
      |       case 'uint8'
      |         dataType = 'fixdt(0,8,0)';
      |       case 'int16'
      |         dataType = 'fixdt(1,16,0)';
      |       case 'uint16'
      |         dataType = 'fixdt(0,16,0)';
      |       case 'int32'
      |         dataType = 'fixdt(1,32,0)';
      |       case 'uint32'
      |         dataType = 'fixdt(0,32,0)';
      |       case 'Specify via dialog'
      |         dataType = OutDataType;
      |     end
      |     
      |     set_param(propBlk, 'PropDataTypeMode', 'Specify via dialog', ...
      |                        'PropScalingMode',  'Specify via dialog', ...
      |                        'PropDataType',     dataType, ...
      |                        'PropScaling',      scaling);
      | end
  id_ref1 : Constant  Value=100  OutDataType=fixdt(1, 16)  OutScaling=2^0
  id_ref2 : Constant  Value=0  OutDataType=fixdt(1, 16)  OutScaling=2^0
  id_ref4 : Constant  Value=-Imax  OutDataType=fixdt(1, 16)  OutScaling=2^0
  id_ref : Outport
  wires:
  id_ref1/1 -> Add3/1
  us/1 -> Add3/2, Compare To Constant/1
  Add/1 -> Saturation Dynamic/2(u)
  Add3/1 -> P2/1, I/1
  id_ref2/1 -> Saturation Dynamic/1(up)
  id_ref4/1 -> Saturation Dynamic/3(lo)
  Compare To Constant/1 -> Integrator1/2
  Saturation Dynamic/1(y1) -> id_ref/1
  I/1 -> Integrator1/1
  P2/1 -> Add/1
  Integrator1/1 -> Add/2
  id_mtpa/1 -> Integrator1/3

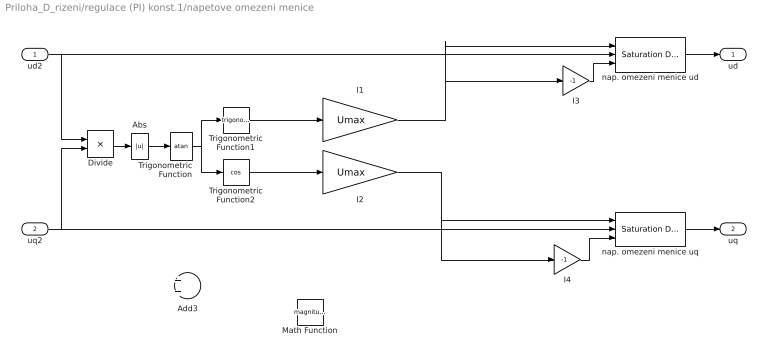
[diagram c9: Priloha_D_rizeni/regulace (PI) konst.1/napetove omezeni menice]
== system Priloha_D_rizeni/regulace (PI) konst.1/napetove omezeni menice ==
  ud2 : Inport
  uq2 : Inport  Port=2
  Abs : Abs  OutDataType=fixdt(1, 16)  OutScaling=2^0
  Add3 : Sum  OutDataType=fixdt(1, 16)  OutScaling=2^-10
  Divide : Product  Inputs=*/  OutDataType=fixdt(1, 16)  OutScaling=2^-10
  I1 : Gain  Gain=Umax  ParameterDataType=fixdt(1, 16)  ParameterScaling=2^0  OutDataType=fixdt(1, 16)  OutScaling=2^0
  I2 : Gain  Gain=Umax  ParameterDataType=fixdt(1, 16)  ParameterScaling=2^0  OutDataType=fixdt(1, 16)  OutScaling=2^0
  I3 : Gain  Gain=-1  ParameterDataType=fixdt(1, 16)  ParameterScaling=2^0  OutDataType=fixdt(1, 16)  OutScaling=2^0
  I4 : Gain  Gain=-1  ParameterDataType=fixdt(1, 16)  ParameterScaling=2^0  OutDataType=fixdt(1, 16)  OutScaling=2^0
  Math Function : Math  Operator=magnitude^2  OutputSignalType=real  OutDataType=fixdt(1, 16)  OutScaling=2^0
  Trigonometric Function : Trigonometry  Operator=atan
  Trigonometric Function1 : Trigonometry
  Trigonometric Function2 : Trigonometry  Operator=cos
  nap. omezeni menice ud : simulink/Discontinuities/Saturation Dynamic  SystemSampleTime=-1  OutMin=[]  OutMax=[]  OutDataTypeStr=Inherit: Same as second input  OutDataType=fixdt(1, 16)  OutScaling=2^-10  DoSatur=off
  nap. omezeni menice uq : simulink/Discontinuities/Saturation Dynamic  SystemSampleTime=-1  OutMin=[]  OutMax=[]  OutDataTypeStr=Inherit: Same as second input  OutDataType=fixdt(1, 16)  OutScaling=2^-10  DoSatur=off
  ud : Outport
  uq : Outport  Port=2
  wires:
  nap. omezeni menice ud/1 -> ud/1
  nap. omezeni menice uq/1 -> uq/1
  ud2/1 -> nap. omezeni menice ud/2, Divide/1
  uq2/1 -> nap. omezeni menice uq/2, Divide/2
  Divide/1 -> Abs/1
  Trigonometric Function/1 -> Trigonometric Function1/1, Trigonometric Function2/1
  Trigonometric Function2/1 -> I2/1
  Trigonometric Function1/1 -> I1/1
  I4/1 -> nap. omezeni menice uq/3
  I2/1 -> I4/1, nap. omezeni menice uq/1
  I3/1 -> nap. omezeni menice ud/3
  I1/1 -> I3/1, nap. omezeni menice ud/1
  Abs/1 -> Trigonometric Function/1

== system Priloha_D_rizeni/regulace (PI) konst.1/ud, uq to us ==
  ud2 : Inport
  uq2 : Inport  Port=2
  Add3 : Sum  OutDataType=fixdt(1, 16)  OutScaling=2^-10
  Math Function : Math  Operator=magnitude^2  OutputSignalType=real  OutDataType=fixdt(1, 16)  OutScaling=2^0
  Math Function1 : Math  Operator=magnitude^2  OutputSignalType=real  OutDataType=fixdt(1, 16)  OutScaling=2^0
  Math Funtion2 : Math  Operator=sqrt  OutputSignalType=real  OutDataType=fixdt(1, 16)  OutScaling=2^0
  us : Outport
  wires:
  Math Function/1 -> Add3/1
  Math Function1/1 -> Add3/2
  Add3/1 -> Math Funtion2/1
  ud2/1 -> Math Function/1
  Math Funtion2/1 -> us/1
  uq2/1 -> Math Function1/1

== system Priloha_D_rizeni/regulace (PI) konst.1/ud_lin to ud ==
  ud1 : Inport
  wm : Inport  Port=2
  iq : Inport  Port=3
  Add6 : Sum  Inputs=+-  OutDataType=fixdt(1, 16)  OutScaling=2^-10
  Gain1 : Gain  Gain=p  ParameterDataType=fixdt(1, 16)  ParameterScaling=2^0  OutDataType=fixdt(1, 16)  OutScaling=2^0
  Gain2 : Gain  Gain=Lq  ParameterDataType=fixdt(1, 16)  ParameterScaling=2^0  OutDataType=fixdt(1, 16)  OutScaling=2^0
  Product6 : Product  OutDataType=fixdt(1, 16)  OutScaling=2^0
  ud2 : Outport
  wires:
  Gain1/1 -> Product6/1
  Product6/1 -> Add6/2
  Add6/1 -> ud2/1
  wm/1 -> Gain1/1
  ud1/1 -> Add6/1
  Gain2/1 -> Product6/2
  iq/1 -> Gain2/1

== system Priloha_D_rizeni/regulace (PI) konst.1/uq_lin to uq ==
  uq1 : Inport
  wm : Inport  Port=2
  id : Inport  Port=3
  Add1 : Sum  OutDataType=fixdt(1, 16)  OutScaling=2^-10
  Add2 : Sum  OutDataType=fixdt(1, 16)  OutScaling=2^-10
  Gain1 : Gain  Gain=Ld  ParameterDataType=fixdt(1, 16)  ParameterScaling=2^0  OutDataType=fixdt(1, 16)  OutScaling=2^0
  Gain2 : Gain  Gain=p  ParameterDataType=fixdt(1, 16)  ParameterScaling=2^0  OutDataType=fixdt(1, 16)  OutScaling=2^0
  Product1 : Product  OutDataType=fixdt(1, 16)  OutScaling=2^0
  id_ref1 : Constant  Value=Ld * Im  OutDataType=fixdt(1, 16)  OutScaling=2^0
  uq2 : Outport
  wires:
  Product1/1 -> Add1/2
  Gain2/1 -> Product1/1
  Add1/1 -> uq2/1
  wm/1 -> Gain2/1
  uq1/1 -> Add1/1
  Add2/1 -> Product1/2
  id/1 -> Gain1/1
  Gain1/1 -> Add2/1
  id_ref1/1 -> Add2/2

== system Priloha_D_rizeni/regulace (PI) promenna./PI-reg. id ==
  note: PI-regulator proudu id
  id_ref : Inport
  id : Inport  Port=2
  Ld : Inport  Port=3
  Add : Sum  OutDataType=fixdt(1, 16)  OutScaling=2^-10
  Add1 : Sum  Inputs=+-  OutDataType=fixdt(1, 16)  OutScaling=2^-10
  Divide : Product  Inputs=**  OutDataType=fixdt(1, 16)  OutScaling=2^-10
  I : Gain  Gain=Kiid  ParameterDataType=fixdt(1, 16)  ParameterScaling=2^0  OutDataType=fixdt(1, 16)  OutScaling=2^0
  Integrator1 : Integrator  LimitOutput=on  UpperSaturationLimit=Umax  LowerSaturationLimit=-Umax
  P2 : Gain  Gain=1 / (KM * 2 * tausigmaid)  ParameterDataType=fixdt(1, 16)  ParameterScaling=2^0  OutDataType=fixdt(1, 16)  OutScaling=2^0
  ud_lin : Outport
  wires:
  P2/1 -> Add/1
  Integrator1/1 -> Add/2
  Add/1 -> ud_lin/1
  id_ref/1 -> Add1/1
  id/1 -> Add1/2
  I/1 -> Integrator1/1
  Add1/1 -> I/1, Divide/2
  Ld/1 -> Divide/1
  Divide/1 -> P2/1

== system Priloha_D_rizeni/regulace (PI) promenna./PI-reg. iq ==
  note: PI-regulator proudu iq
  iq_ref : Inport
  iq : Inport  Port=2
  Lq : Inport  Port=3
  Add : Sum  OutDataType=fixdt(1, 16)  OutScaling=2^-10
  Add1 : Sum  Inputs=+-  OutDataType=fixdt(1, 16)  OutScaling=2^-10
  Divide : Product  Inputs=**  OutDataType=fixdt(1, 16)  OutScaling=2^-10
  I : Gain  Gain=Kiiq  ParameterDataType=fixdt(1, 16)  ParameterScaling=2^0  OutDataType=fixdt(1, 16)  OutScaling=2^0
  Integrator1 : Integrator  LimitOutput=on  UpperSaturationLimit=Umax  LowerSaturationLimit=-Umax
  P : Gain  Gain=1 / (KM * 2 * tausigmaiq)  ParameterDataType=fixdt(1, 16)  ParameterScaling=2^0  OutDataType=fixdt(1, 16)  OutScaling=2^0
  uq_lin : Outport
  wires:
  Integrator1/1 -> Add/2
  P/1 -> Add/1
  Add1/1 -> I/1, Divide/2
  iq_ref/1 -> Add1/1
  iq/1 -> Add1/2
  Add/1 -> uq_lin/1
  I/1 -> Integrator1/1
  Divide/1 -> P/1
  Lq/1 -> Divide/1

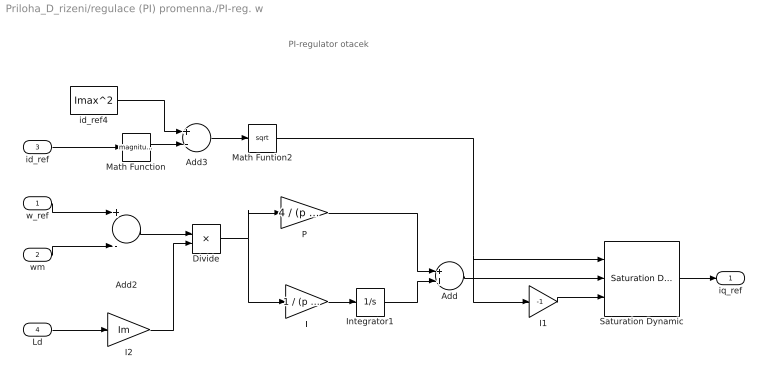
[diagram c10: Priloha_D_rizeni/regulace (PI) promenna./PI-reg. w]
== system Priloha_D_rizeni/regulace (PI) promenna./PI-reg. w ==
  note: PI-regulator otacek
  w_ref : Inport
  wm : Inport  Port=2
  id_ref : Inport  Port=3
  Ld : Inport  Port=4
  Add : Sum  OutDataType=fixdt(1, 16)  OutScaling=2^-10
  Add2 : Sum  Inputs=+-  OutDataType=fixdt(1, 16)  OutScaling=2^-10
  Add3 : Sum  Inputs=+-  OutDataType=fixdt(1, 16)  OutScaling=2^-10
  Divide : Product  Inputs=*/  OutDataType=fixdt(1, 16)  OutScaling=2^-10
  I : Gain  Gain=1 / (p * 8 * (2 * tausigmaiq)^2 / J)  ParameterDataType=fixdt(1, 16)  ParameterScaling=2^0  OutDataType=fixdt(1, 16)  OutScaling=2^0
  I1 : Gain  Gain=-1  ParameterDataType=fixdt(1, 16)  ParameterScaling=2^0  OutDataType=fixdt(1, 16)  OutScaling=2^0
  I2 : Gain  Gain=Im  ParameterDataType=fixdt(1, 16)  ParameterScaling=2^0  OutDataType=fixdt(1, 16)  OutScaling=2^0
  Integrator1 : Integrator  LimitOutput=on  UpperSaturationLimit=Imax  LowerSaturationLimit=-Imax
  Math Function : Math  Operator=magnitude^2  OutputSignalType=real  OutDataType=fixdt(1, 16)  OutScaling=2^0
  Math Funtion2 : Math  Operator=sqrt  OutputSignalType=real  OutDataType=fixdt(1, 16)  OutScaling=2^0
  P : Gain  Gain=4 / (p * 8 * (2 * tausigmaiq) / J)  ParameterDataType=fixdt(1, 16)  ParameterScaling=2^0  OutDataType=fixdt(1, 16)  OutScaling=2^0
  Saturation Dynamic : simulink/Discontinuities/Saturation Dynamic  SystemSampleTime=-1  OutMin=[]  OutMax=[]  OutDataTypeStr=Inherit: Same as second input  OutDataType=fixdt(1, 16)  OutScaling=2^-10  DoSatur=off
  id_ref4 : Constant  Value=Imax^2  OutDataType=fixdt(1, 16)  OutScaling=2^0
  iq_ref : Outport
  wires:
  Add/1 -> Saturation Dynamic/2
  w_ref/1 -> Add2/1
  wm/1 -> Add2/2
  Saturation Dynamic/1 -> iq_ref/1
  I/1 -> Integrator1/1
  id_ref/1 -> Math Function/1
  Add3/1 -> Math Funtion2/1
  Math Funtion2/1 -> Saturation Dynamic/1, I1/1
  Math Function/1 -> Add3/2
  id_ref4/1 -> Add3/1
  I1/1 -> Saturation Dynamic/3
  Integrator1/1 -> Add/2
  P/1 -> Add/1
  Ld/1 -> I2/1
  Add2/1 -> Divide/1
  Divide/1 -> I/1, P/1
  I2/1 -> Divide/2

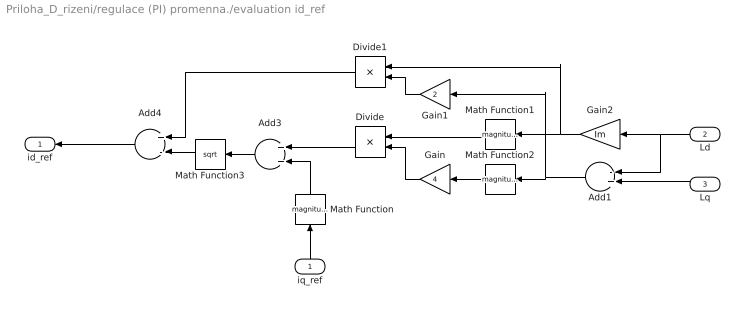
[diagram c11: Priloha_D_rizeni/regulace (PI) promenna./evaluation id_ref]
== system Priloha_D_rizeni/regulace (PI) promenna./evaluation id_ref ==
  iq_ref : Inport
  Ld : Inport  Port=2
  Lq : Inport  Port=3
  Add1 : Sum  Inputs=-+  OutDataType=fixdt(1, 16)  OutScaling=2^-10
  Add3 : Sum  OutDataType=fixdt(1, 16)  OutScaling=2^-10
  Add4 : Sum  Inputs=+-  OutDataType=fixdt(1, 16)  OutScaling=2^-10
  Divide : Product  Inputs=*/  OutDataType=fixdt(1, 16)  OutScaling=2^-10
  Divide1 : Product  Inputs=*/  OutDataType=fixdt(1, 16)  OutScaling=2^-10
  Gain : Gain  Gain=4  ParameterDataType=fixdt(1, 16)  ParameterScaling=2^0  OutDataType=fixdt(1, 16)  OutScaling=2^0
  Gain1 : Gain  Gain=2  ParameterDataType=fixdt(1, 16)  ParameterScaling=2^0  OutDataType=fixdt(1, 16)  OutScaling=2^0
  Gain2 : Gain  Gain=Im  ParameterDataType=fixdt(1, 16)  ParameterScaling=2^0  OutDataType=fixdt(1, 16)  OutScaling=2^0
  Math Function : Math  Operator=magnitude^2  OutputSignalType=real  OutDataType=fixdt(1, 16)  OutScaling=2^0
  Math Function1 : Math  Operator=magnitude^2  OutputSignalType=real  OutDataType=fixdt(1, 16)  OutScaling=2^0
  Math Function2 : Math  Operator=magnitude^2  OutputSignalType=real  OutDataType=fixdt(1, 16)  OutScaling=2^0
  Math Function3 : Math  Operator=sqrt  OutputSignalType=real  OutDataType=fixdt(1, 16)  OutScaling=2^0
  id_ref : Outport
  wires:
  Math Function/1 -> Add3/2
  Gain2/1 -> Math Function1/1, Divide1/1
  Math Function1/1 -> Divide/1
  Math Function2/1 -> Gain/1
  Divide/1 -> Add3/1
  Add3/1 -> Math Function3/1
  Divide1/1 -> Add4/1
  Add1/1 -> Math Function2/1, Gain1/1
  Math Function3/1 -> Add4/2
  Gain/1 -> Divide/2
  Gain1/1 -> Divide1/2
  iq_ref/1 -> Math Function/1
  Add4/1 -> id_ref/1
  Ld/1 -> Gain2/1, Add1/1
  Lq/1 -> Add1/2

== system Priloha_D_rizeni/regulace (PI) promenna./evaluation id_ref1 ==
  iq_ref : Inport
  Add3 : Sum  OutDataType=fixdt(1, 16)  OutScaling=2^-10
  Add4 : Sum  Inputs=+-  OutDataType=fixdt(1, 16)  OutScaling=2^-10
  Divide : Product  Inputs=*/  OutDataType=fixdt(1, 16)  OutScaling=2^-10
  Divide1 : Product  Inputs=*/  OutDataType=fixdt(1, 16)  OutScaling=2^-10
  Gain : Gain  Gain=4  ParameterDataType=fixdt(1, 16)  ParameterScaling=2^0  OutDataType=fixdt(1, 16)  OutScaling=2^0
  Gain1 : Gain  Gain=2  ParameterDataType=fixdt(1, 16)  ParameterScaling=2^0  OutDataType=fixdt(1, 16)  OutScaling=2^0
  Math Function : Math  Operator=magnitude^2  OutputSignalType=real  OutDataType=fixdt(1, 16)  OutScaling=2^0
  Math Function1 : Math  Operator=magnitude^2  OutputSignalType=real  OutDataType=fixdt(1, 16)  OutScaling=2^0
  Math Function2 : Math  Operator=magnitude^2  OutputSignalType=real  OutDataType=fixdt(1, 16)  OutScaling=2^0
  Math Function3 : Math  Operator=sqrt  OutputSignalType=real  OutDataType=fixdt(1, 16)  OutScaling=2^0
  w_ref1 : Constant  Value=Lq - Ld  OutDataType=fixdt(1, 16)  OutScaling=2^0
  w_ref2 : Constant  Value=Psim  OutDataType=fixdt(1, 16)  OutScaling=2^0
  id_ref : Outport
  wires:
  Math Function/1 -> Add3/2
  w_ref2/1 -> Math Function1/1, Divide1/1
  Math Function1/1 -> Divide/1
  Math Function2/1 -> Gain/1
  Divide/1 -> Add3/1
  Add3/1 -> Math Function3/1
  Divide1/1 -> Add4/1
  w_ref1/1 -> Math Function2/1, Gain1/1
  Math Function3/1 -> Add4/2
  Gain/1 -> Divide/2
  Gain1/1 -> Divide1/2
  iq_ref/1 -> Math Function/1
  Add4/1 -> id_ref/1

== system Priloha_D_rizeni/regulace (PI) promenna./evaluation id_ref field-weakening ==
  note: PI-regulator napeti
  us : Inport
  id_mtpa : Inport  Port=2
  Add : Sum  OutDataType=fixdt(1, 16)  OutScaling=2^-10
  Add3 : Sum  Inputs=+-  OutDataType=fixdt(1, 16)  OutScaling=2^-10
  Compare To Constant : simulink/Logic and Bit Operations/Compare To Constant  SystemSampleTime=-1  relop=<  const=Umax * 0.98  LogicOutDataTypeMode=boolean
  I : Gain  Gain=10  ParameterDataType=fixdt(1, 16)  ParameterScaling=2^0  OutDataType=fixdt(1, 16)  OutScaling=2^0
  Integrator1 : Integrator  ExternalReset=level  InitialConditionSource=external  LimitOutput=on  UpperSaturationLimit=Imax  LowerSaturationLimit=-Imax
  P2 : Gain  Gain=0.08  ParameterDataType=fixdt(1, 16)  ParameterScaling=2^0  OutDataType=fixdt(1, 16)  OutScaling=2^0
  Saturation Dynamic : simulink/Discontinuities/Saturation Dynamic  SystemSampleTime=-1  OutMin=[]  OutMax=[]  OutDataTypeStr=Inherit: Same as second input  OutDataType=fixdt(1, 16)  OutScaling=2^-10  DoSatur=off
  id_ref1 : Constant  Value=100  OutDataType=fixdt(1, 16)  OutScaling=2^0
  id_ref2 : Constant  Value=0  OutDataType=fixdt(1, 16)  OutScaling=2^0
  id_ref4 : Constant  Value=-Imax  OutDataType=fixdt(1, 16)  OutScaling=2^0
  id_ref : Outport
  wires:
  id_ref1/1 -> Add3/1
  us/1 -> Add3/2, Compare To Constant/1
  Add/1 -> Saturation Dynamic/2
  Add3/1 -> P2/1, I/1
  id_ref2/1 -> Saturation Dynamic/1
  id_ref4/1 -> Saturation Dynamic/3
  Compare To Constant/1 -> Integrator1/2
  Saturation Dynamic/1 -> id_ref/1
  I/1 -> Integrator1/1
  id_mtpa/1 -> Integrator1/3
  Integrator1/1 -> Add/2
  P2/1 -> Add/1

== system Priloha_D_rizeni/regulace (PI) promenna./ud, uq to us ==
  ud : Inport
  uq : Inport  Port=2
  Add3 : Sum  OutDataType=fixdt(1, 16)  OutScaling=2^-10
  Math Function : Math  Operator=magnitude^2  OutputSignalType=real  OutDataType=fixdt(1, 16)  OutScaling=2^0
  Math Function1 : Math  Operator=magnitude^2  OutputSignalType=real  OutDataType=fixdt(1, 16)  OutScaling=2^0
  Math Funtion2 : Math  Operator=sqrt  OutputSignalType=real  OutDataType=fixdt(1, 16)  OutScaling=2^0
  us : Outport
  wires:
  Math Function/1 -> Add3/1
  Math Function1/1 -> Add3/2
  Add3/1 -> Math Funtion2/1
  ud/1 -> Math Function/1
  Math Funtion2/1 -> us/1
  uq/1 -> Math Function1/1

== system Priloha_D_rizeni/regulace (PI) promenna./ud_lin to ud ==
  ud_lin : Inport
  wm : Inport  Port=2
  iq : Inport  Port=3
  Lq : Inport  Port=4
  Add6 : Sum  Inputs=+-  OutDataType=fixdt(1, 16)  OutScaling=2^-10
  Divide : Product  Inputs=**  OutDataType=fixdt(1, 16)  OutScaling=2^-10
  Gain1 : Gain  Gain=p  ParameterDataType=fixdt(1, 16)  ParameterScaling=2^0  OutDataType=fixdt(1, 16)  OutScaling=2^0
  Product6 : Product  OutDataType=fixdt(1, 16)  OutScaling=2^0
  ud1 : Outport
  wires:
  Gain1/1 -> Product6/1
  Product6/1 -> Add6/2
  Add6/1 -> ud1/1
  wm/1 -> Gain1/1
  ud_lin/1 -> Add6/1
  iq/1 -> Divide/1
  Divide/1 -> Product6/2
  Lq/1 -> Divide/2

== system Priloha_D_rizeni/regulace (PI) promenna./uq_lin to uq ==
  uq_lin : Inport
  wm : Inport  Port=2
  id : Inport  Port=3
  Ld : Inport  Port=4
  Add1 : Sum  OutDataType=fixdt(1, 16)  OutScaling=2^-10
  Add2 : Sum  OutDataType=fixdt(1, 16)  OutScaling=2^-10
  Divide : Product  Inputs=**  OutDataType=fixdt(1, 16)  OutScaling=2^-10
  Gain1 : Gain  Gain=Im  ParameterDataType=fixdt(1, 16)  ParameterScaling=2^0  OutDataType=fixdt(1, 16)  OutScaling=2^0
  Gain2 : Gain  Gain=p  ParameterDataType=fixdt(1, 16)  ParameterScaling=2^0  OutDataType=fixdt(1, 16)  OutScaling=2^0
  Product1 : Product  OutDataType=fixdt(1, 16)  OutScaling=2^0
  uq1 : Outport
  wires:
  Product1/1 -> Add1/2
  Gain2/1 -> Product1/1
  Add1/1 -> uq1/1
  wm/1 -> Gain2/1
  uq_lin/1 -> Add1/1
  Add2/1 -> Product1/2
  Divide/1 -> Add2/1
  id/1 -> Divide/1
  Ld/1 -> Divide/2, Gain1/1
  Gain1/1 -> Add2/2

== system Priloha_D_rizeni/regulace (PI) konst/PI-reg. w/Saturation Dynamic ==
  up : Inport  OutDataType=fixdt(1, 16)  OutScaling=2^0
  u : Inport  Port=2  OutDataType=fixdt(1, 16)  OutScaling=2^0
  lo : Inport  Port=3  OutDataType=fixdt(1, 16)  OutScaling=2^0
  Data Type Duplicate : simulink/Signal Attributes/Data Type Duplicate  NumInputPorts=2
  Data Type Propagation : simulink/Signal Attributes/Data Type Propagation  PropDataType=fixdt(1, 16)  IfRefDouble=double  IfRefSingle=single  IsSigned=IsSigned1  NumBitsBase=NumBits1  NumBitsMult=1  NumBitsAdd=0  NumBitsAllowFinal=1:128  PropScaling=2^-10  ValuesUsedBestPrec=[5 -7]  SlopeBase=Slope1  SlopeMult=1  SlopeAdd=0  BiasBase=Bias1  BiasMult=1  BiasAdd=0
  LowerRelop1 : RelationalOperator  DisableCoverage=on  Operator=>  LogicOutDataTypeMode=boolean  LogicDataType=fixdt(0, 8)  OutDataTypeStr=boolean
  Switch : Switch  Criteria=u2 ~= 0  OutDataType=fixdt(1, 16)  OutScaling=2^0  OutDataTypeStr=Inherit: Inherit via back propagation  ZeroCross=off
  Switch2 : Switch  Criteria=u2 ~= 0  OutMin=OutMin  OutMax=OutMax  OutDataType=OutDataType  OutScaling=OutScaling  OutDataTypeStr=Inherit: Inherit via back propagation  ZeroCross=off
  UpperRelop : RelationalOperator  DisableCoverage=on  Operator=<  LogicOutDataTypeMode=boolean  LogicDataType=fixdt(0, 8)  OutDataTypeStr=boolean
  y1 : Outport  OutMin=OutMin  OutMax=OutMax  OutDataType=fixdt(1, 16)  OutScaling=2^0
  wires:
  up/1 -> Switch2/1, LowerRelop1/2
  u/1 -> Data Type Propagation/2, Data Type Propagation/1, LowerRelop1/1, Switch/3, UpperRelop/1
  lo/1 -> Switch/1, UpperRelop/2
  Switch/1 -> Data Type Duplicate/2, Switch2/3, Data Type Propagation/3
  Switch2/1 -> Data Type Duplicate/1, y1/1
  LowerRelop1/1 -> Switch2/2
  UpperRelop/1 -> Switch/2
